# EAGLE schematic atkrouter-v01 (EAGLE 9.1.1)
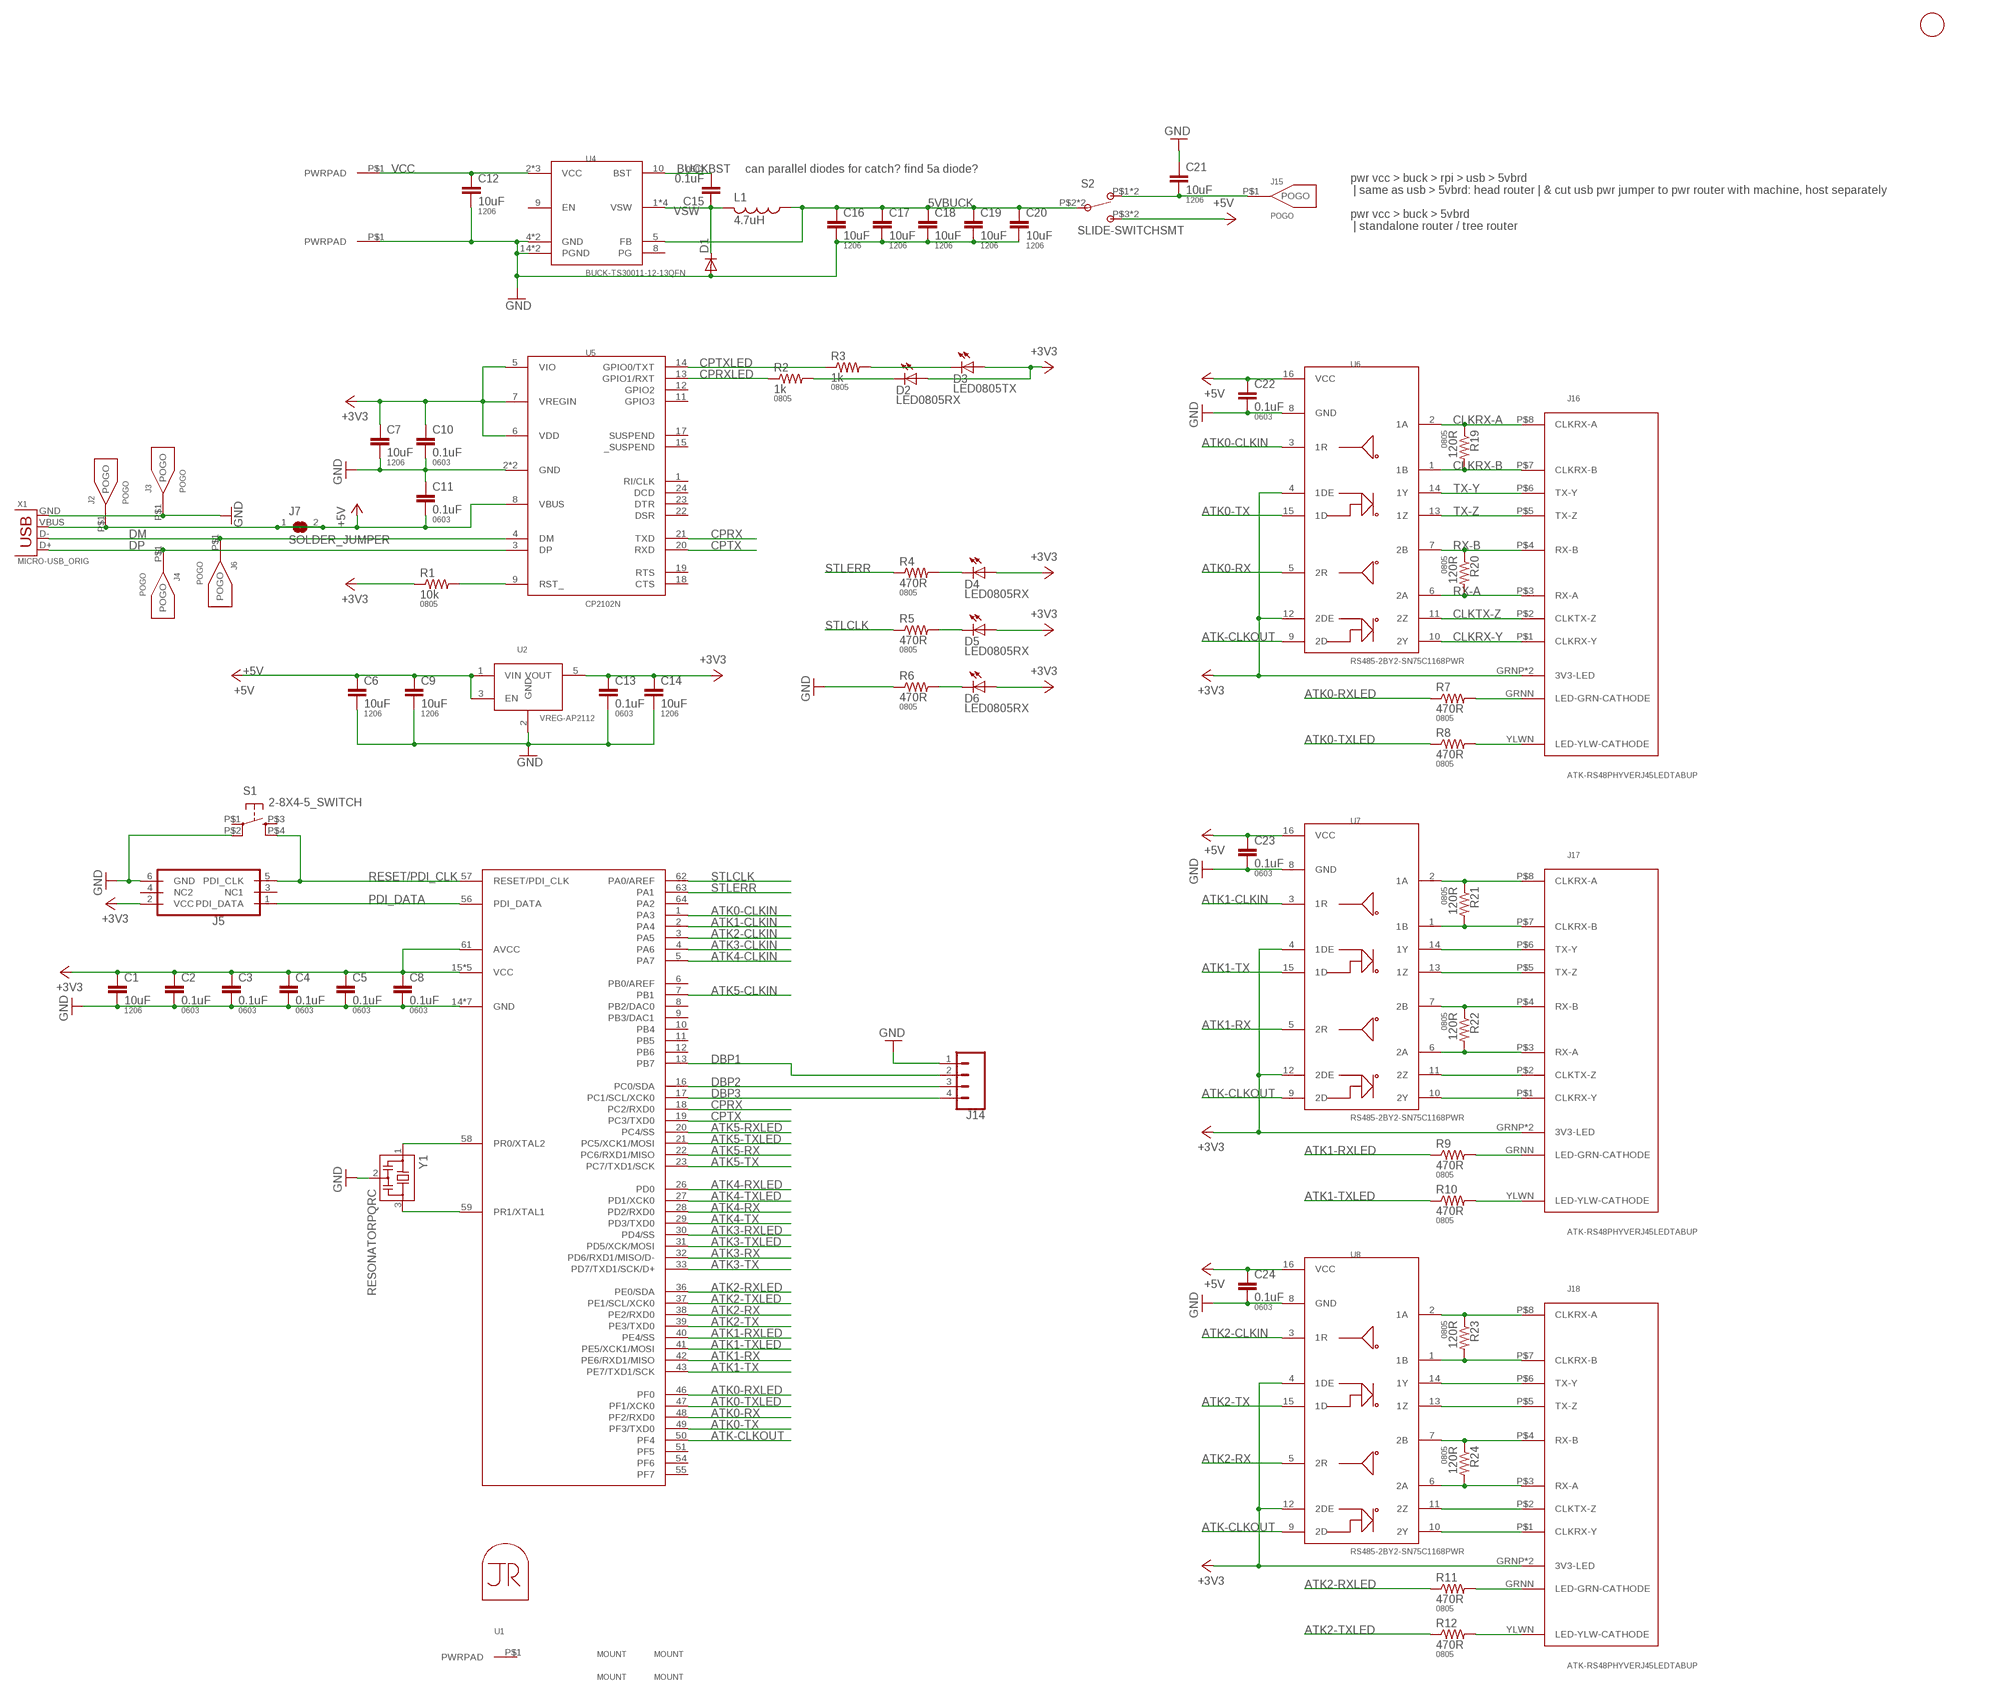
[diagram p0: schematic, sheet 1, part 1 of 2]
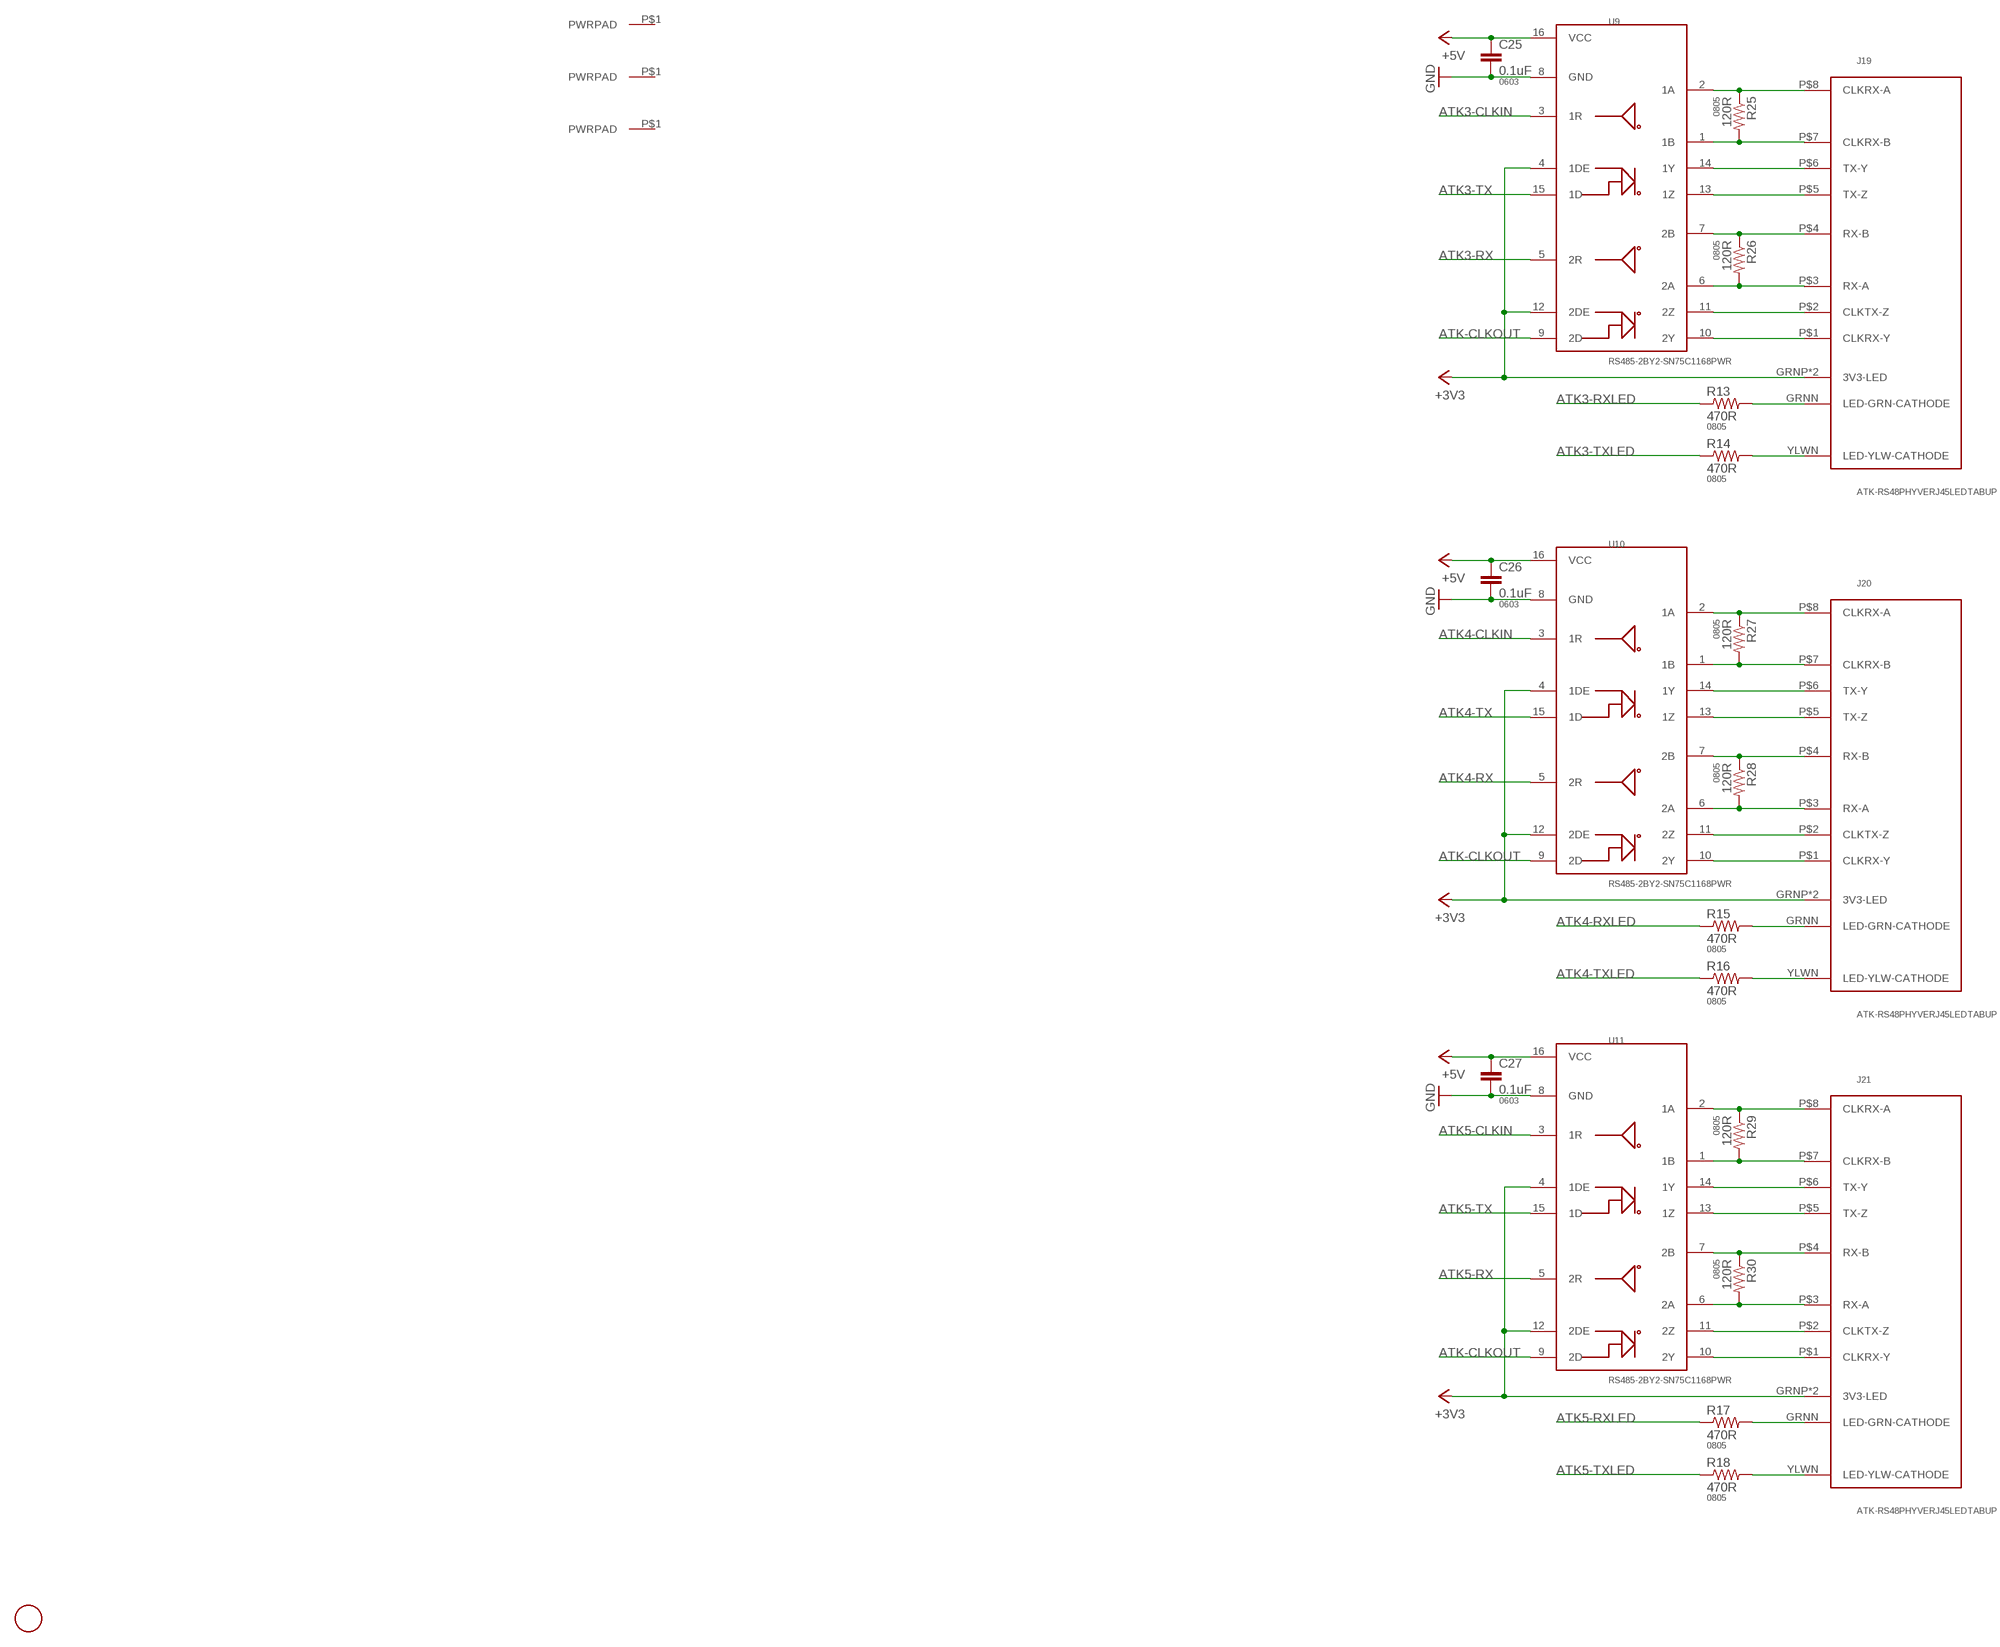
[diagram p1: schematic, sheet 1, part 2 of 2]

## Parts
C1  10uF  CAP1206  [1206]
C2  0.1uF  CAP0603-CAP  [0603-CAP]
C3  0.1uF  CAP0603-CAP  [0603-CAP]
C4  0.1uF  CAP0603-CAP  [0603-CAP]
C5  0.1uF  CAP0603-CAP  [0603-CAP]
C6  10uF  CAP1206  [1206]
C7  10uF  CAP1206  [1206]
C8  0.1uF  CAP0603-CAP  [0603-CAP]
C9  10uF  CAP1206  [1206]
C10  0.1uF  CAP0603-CAP  [0603-CAP]
C11  0.1uF  CAP0603-CAP  [0603-CAP]
C12  10uF  CAP1206  [1206]
C13  0.1uF  CAP0603-CAP  [0603-CAP]
C14  10uF  CAP1206  [1206]
C15  0.1uF  CAP0603-CAP  [0603-CAP]
C16  10uF  CAP1206  [1206]
C17  10uF  CAP1206  [1206]
C18  10uF  CAP1206  [1206]
C19  10uF  CAP1206  [1206]
C20  10uF  CAP1206  [1206]
C21  10uF  CAP1206  [1206]
C22  0.1uF  CAP0603-CAP  [0603-CAP]
C23  0.1uF  CAP0603-CAP  [0603-CAP]
C24  0.1uF  CAP0603-CAP  [0603-CAP]
C25  0.1uF  CAP0603-CAP  [0603-CAP]
C26  0.1uF  CAP0603-CAP  [0603-CAP]
C27  0.1uF  CAP0603-CAP  [0603-CAP]
D1  DIODESOD123HE  [SOD-123HE]
D2  LED0805RX  LED0805  [LED0805]
D3  LED0805TX  LED0805  [LED0805]
D4  LED0805RX  LED0805  [LED0805]
D5  LED0805RX  LED0805  [LED0805]
D6  LED0805RX  LED0805  [LED0805]
J1  FIDUCIAL  [FIDUCIAL_1MM]
J2  POGO  [POGO]
J3  POGO  [POGO]
J4  POGO  [POGO]
J5  PDIFEMALE_SMD  [PDI_2X3_SMD]
J6  POGO  [POGO]
J7  SOLDER_JUMPER  [SJFAB]
J8  PWRPADM3-STANDOFF  [PWRPAD_M3_STANDOFF]
J9  PWRPADM3-STANDOFF  [PWRPAD_M3_STANDOFF]
J10  PWRPADM2.5_STANDOFF  [PWRPAD_M25_STANDOFF]
J11  PWRPADM2.5_STANDOFF  [PWRPAD_M25_STANDOFF]
J12  PWRPADM2.5_STANDOFF  [PWRPAD_M25_STANDOFF]
J13  PWRPADM2.5_STANDOFF  [PWRPAD_M25_STANDOFF]
J14  CONN_041X04_NO_SILK  [1X04_NO_SILK]
J15  POGO  [POGO]
J16  ATK-RS48PHYVERJ45LEDTABUP  [RJ45-LED-RJHSE-5381-UPTAB]
J17  ATK-RS48PHYVERJ45LEDTABUP  [RJ45-LED-RJHSE-5381-UPTAB]
J18  ATK-RS48PHYVERJ45LEDTABUP  [RJ45-LED-RJHSE-5381-UPTAB]
J19  ATK-RS48PHYVERJ45LEDTABUP  [RJ45-LED-RJHSE-5381-UPTAB]
J20  ATK-RS48PHYVERJ45LEDTABUP  [RJ45-LED-RJHSE-5381-UPTAB]
J21  ATK-RS48PHYVERJ45LEDTABUP  [RJ45-LED-RJHSE-5381-UPTAB]
J22  FIDUCIAL  [FIDUCIAL_1MM]
L1  4.7uH  INDUCTOR  [NRS5020T4R7MMGJ]
M1  M3-NPTH  [NPTH-3-25MM]
M2  M3-NPTH  [NPTH-3-25MM]
M3  M3-NPTH  [NPTH-3-25MM]
M4  M3-NPTH  [NPTH-3-25MM]
MP1  JRTOMBSTONE  [JRTOMBSTONE]
R1  10k  RESISTOR0805-RES  [0805]
R2  1k  RESISTOR0805-RES  [0805]
R3  1k  RESISTOR0805-RES  [0805]
R4  470R  RESISTOR0805-RES  [0805]
R5  470R  RESISTOR0805-RES  [0805]
R6  470R  RESISTOR0805-RES  [0805]
R7  470R  RESISTOR0805-RES  [0805]
R8  470R  RESISTOR0805-RES  [0805]
R9  470R  RESISTOR0805-RES  [0805]
R10  470R  RESISTOR0805-RES  [0805]
R11  470R  RESISTOR0805-RES  [0805]
R12  470R  RESISTOR0805-RES  [0805]
R13  470R  RESISTOR0805-RES  [0805]
R14  470R  RESISTOR0805-RES  [0805]
R15  470R  RESISTOR0805-RES  [0805]
R16  470R  RESISTOR0805-RES  [0805]
R17  470R  RESISTOR0805-RES  [0805]
R18  470R  RESISTOR0805-RES  [0805]
R19  120R  RESISTOR0805-RES  [0805]
R20  120R  RESISTOR0805-RES  [0805]
R21  120R  RESISTOR0805-RES  [0805]
R22  120R  RESISTOR0805-RES  [0805]
R23  120R  RESISTOR0805-RES  [0805]
R24  120R  RESISTOR0805-RES  [0805]
R25  120R  RESISTOR0805-RES  [0805]
R26  120R  RESISTOR0805-RES  [0805]
R27  120R  RESISTOR0805-RES  [0805]
R28  120R  RESISTOR0805-RES  [0805]
R29  120R  RESISTOR0805-RES  [0805]
R30  120R  RESISTOR0805-RES  [0805]
S1  2-8X4-5_SWITCH  [TACT-SWITCH-KMR6]
S2  SLIDE-SWITCHSMT  [SLIDESWITCH-CL-SB-22A]
U1  RASPBERRYPI-3BPLUS  [RASPBERRYPI-3BPLUS]
U2  VREG-AP2112  [SOT23-5]
U3  ATXMEGA_A3UQFN  [QFN-64-9X9MM]
U4  BUCK-TS30011-12-13QFN  [QFN16-3X3-TI-RTE]
U5  CP2102N  [QFN-24_ALT2]
U6  RS485-2BY2-SN75C1168PWR  [TSSOP16]
U7  RS485-2BY2-SN75C1168PWR  [TSSOP16]
U8  RS485-2BY2-SN75C1168PWR  [TSSOP16]
U9  RS485-2BY2-SN75C1168PWR  [TSSOP16]
U10  RS485-2BY2-SN75C1168PWR  [TSSOP16]
U11  RS485-2BY2-SN75C1168PWR  [TSSOP16]
X1  MICRO-USB_ORIG  [DX4R005HJ5]
Y1  RESONATORPQRC  [RES_PRQC]

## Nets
5VBUCK: C16.1 C17.1 C18.1 C19.1 C20.1 L1.1 S2.P$2 S2.P$5 U4.5(FB)
+3V3: C1.1 C2.1 C3.1 C4.1 C5.1 C7.1 C8.1 C10.1 C13.1 C14.1 D2.1(A) D3.1(A) D4.1(A) D5.1(A) D6.1(A) J5.2(VCC) J16.GRNP(3V3-LED) J16.YLWP(3V3-LED) J17.GRNP(3V3-LED) J17.YLWP(3V3-LED) J18.GRNP(3V3-LED) J18.YLWP(3V3-LED) J19.GRNP(3V3-LED) J19.YLWP(3V3-LED) J20.GRNP(3V3-LED) J20.YLWP(3V3-LED) J21.GRNP(3V3-LED) J21.YLWP(3V3-LED) R1.1 U2.5(VOUT) U3.15(VCC) U3.25(VCC) U3.35(VCC) U3.45(VCC) U3.53(VCC) U3.61(AVCC) U5.5(VIO) U5.6(VDD) U5.7(VREGIN) U6.4(1DE) U6.12(2DE) U7.4(1DE) U7.12(2DE) U8.4(1DE) U8.12(2DE) U9.4(1DE) U9.12(2DE) U10.4(1DE) U10.12(2DE) U11.4(1DE) U11.12(2DE)
+5V: C6.1 C9.1 C11.2 C22.1 C23.1 C24.1 C25.1 C26.1 C27.1 J2.P$1(POGO) J7.1 J7.2 S2.P$3 S2.P$6 U2.1(VIN) U2.3(EN) U5.8(VBUS) U6.16(VCC) U7.16(VCC) U8.16(VCC) U9.16(VCC) U10.16(VCC) U11.16(VCC) X1.VBUS
ATK0-CLKIN: U3.1(PA3) U6.3(1R)
ATK0-RX: U3.48(PF2/RXD0) U6.5(2R)
ATK0-RXLED: R7.1 U3.46(PF0)
ATK0-TX: U3.49(PF3/TXD0) U6.15(1D)
ATK0-TXLED: R8.1 U3.47(PF1/XCK0)
ATK1-CLKIN: U3.2(PA4) U7.3(1R)
ATK1-RX: U3.42(PE6/RXD1/MISO) U7.5(2R)
ATK1-RXLED: R9.1 U3.40(PE4/SS)
ATK1-TX: U3.43(PE7/TXD1/SCK) U7.15(1D)
ATK1-TXLED: R10.1 U3.41(PE5/XCK1/MOSI)
ATK2-CLKIN: U3.3(PA5) U8.3(1R)
ATK2-RX: U3.38(PE2/RXD0) U8.5(2R)
ATK2-RXLED: R11.1 U3.36(PE0/SDA)
ATK2-TX: U3.39(PE3/TXD0) U8.15(1D)
ATK2-TXLED: R12.1 U3.37(PE1/SCL/XCK0)
ATK3-CLKIN: U3.4(PA6) U9.3(1R)
ATK3-RX: U3.32(PD6/RXD1/MISO/D-) U9.5(2R)
ATK3-RXLED: R13.1 U3.30(PD4/SS)
ATK3-TX: U3.33(PD7/TXD1/SCK/D+) U9.15(1D)
ATK3-TXLED: R14.1 U3.31(PD5/XCK/MOSI)
ATK4-CLKIN: U3.5(PA7) U10.3(1R)
ATK4-RX: U3.28(PD2/RXD0) U10.5(2R)
ATK4-RXLED: R15.1 U3.26(PD0)
ATK4-TX: U3.29(PD3/TXD0) U10.15(1D)
ATK4-TXLED: R16.1 U3.27(PD1/XCK0)
ATK5-CLKIN: U3.7(PB1) U11.3(1R)
ATK5-RX: U3.22(PC6/RXD1/MISO) U11.5(2R)
ATK5-RXLED: R17.1 U3.20(PC4/SS)
ATK5-TX: U3.23(PC7/TXD1/SCK) U11.15(1D)
ATK5-TXLED: R18.1 U3.21(PC5/XCK1/MOSI)
ATK-CLKOUT: U3.50(PF4) U6.9(2D) U7.9(2D) U8.9(2D) U9.9(2D) U10.9(2D) U11.9(2D)
BUCKBST: C15.2 U4.10(BST)
CLKRX-A: J16.P$8(CLKRX-A) R19.1 U6.2(1A)
CLKRX-B: J16.P$7(CLKRX-B) R19.2 U6.1(1B)
CLKRX-Y: J16.P$1(CLKRX-Y) U6.10(2Y)
CLKTX-Z: J16.P$2(CLKTX-Z) U6.11(2Z)
CPRX: U3.18(PC2/RXD0) U5.21(TXD)
CPRXLED: R2.1 U5.13(GPIO1/RXT)
CPTX: U3.19(PC3/TXD0) U5.20(RXD)
CPTXLED: R3.1 U5.14(GPIO0/TXT)
DBP1: J14.2 U3.13(PB7)
DBP2: J14.3 U3.16(PC0/SDA)
DBP3: J14.4 U3.17(PC1/SCL/XCK0)
DM: J6.P$1(POGO) U5.4(DM) X1.D-
DP: J4.P$1(POGO) U5.3(DP) X1.D+
GND: C1.2 C2.2 C3.2 C4.2 C5.2 C6.2 C7.2 C8.2 C9.2 C10.2 C11.1 C12.2 C13.2 C14.2 C16.2 C17.2 C18.2 C19.2 C20.2 C21.1 C22.2 C23.2 C24.2 C25.2 C26.2 C27.2 D1.P$2(A) J3.P$1(POGO) J5.6(GND) J9.P$1(PWRPAD) J14.1 R6.1 S1.P$2(P1) U2.2(GND) U3.14(GND) U3.24(GND) U3.34(GND) U3.44(GND) U3.52(GND) U3.60(GND) U3.P$1(GND) U4.4(GND) U4.14(PGND) U4.15(PGND) U4.TH(GND) U5.2(GND) U5.EP(GND) U6.8(GND) U7.8(GND) U8.8(GND) U9.8(GND) U10.8(GND) U11.8(GND) X1.GND Y1.2
N$1: J16.GRNN(LED-GRN-CATHODE) R7.2
N$2: J16.YLWN(LED-YLW-CATHODE) R8.2
N$3: J18.P$6(TX-Y) U8.14(1Y)
N$4: J18.P$5(TX-Z) U8.13(1Z)
N$5: J18.P$4(RX-B) R24.1 U8.7(2B)
N$6: J18.P$3(RX-A) R24.2 U8.6(2A)
N$7: J18.P$8(CLKRX-A) R23.1 U8.2(1A)
N$8: J18.P$7(CLKRX-B) R23.2 U8.1(1B)
N$9: J18.P$2(CLKTX-Z) U8.11(2Z)
N$10: J18.P$1(CLKRX-Y) U8.10(2Y)
N$13: U3.58(PR0/XTAL2) Y1.1
N$14: U3.59(PR1/XTAL1) Y1.3
N$15: D6.2(C) R6.2
N$17: D5.2(C) R5.2
N$19: R1.2 U5.9(RST_)
N$21: D4.2(C) R4.2
N$25: J17.P$6(TX-Y) U7.14(1Y)
N$26: J17.P$5(TX-Z) U7.13(1Z)
N$27: J17.P$4(RX-B) R22.1 U7.7(2B)
N$28: J17.P$3(RX-A) R22.2 U7.6(2A)
N$29: J17.P$8(CLKRX-A) R21.1 U7.2(1A)
N$30: J17.P$7(CLKRX-B) R21.2 U7.1(1B)
N$31: J17.P$2(CLKTX-Z) U7.11(2Z)
N$32: J17.P$1(CLKRX-Y) U7.10(2Y)
N$33: J17.GRNN(LED-GRN-CATHODE) R9.2
N$34: J17.YLWN(LED-YLW-CATHODE) R10.2
N$35: J18.GRNN(LED-GRN-CATHODE) R11.2
N$36: J18.YLWN(LED-YLW-CATHODE) R12.2
N$37: D2.2(C) R2.2
N$38: D3.2(C) R3.2
N$39: J19.P$6(TX-Y) U9.14(1Y)
N$40: J19.P$5(TX-Z) U9.13(1Z)
N$41: J19.P$4(RX-B) R26.1 U9.7(2B)
N$42: J19.P$3(RX-A) R26.2 U9.6(2A)
N$43: J19.P$8(CLKRX-A) R25.1 U9.2(1A)
N$44: J19.P$7(CLKRX-B) R25.2 U9.1(1B)
N$45: J19.P$2(CLKTX-Z) U9.11(2Z)
N$46: J19.P$1(CLKRX-Y) U9.10(2Y)
N$47: J19.GRNN(LED-GRN-CATHODE) R13.2
N$48: J19.YLWN(LED-YLW-CATHODE) R14.2
N$49: J20.P$6(TX-Y) U10.14(1Y)
N$50: J20.P$5(TX-Z) U10.13(1Z)
N$51: J20.P$4(RX-B) R28.1 U10.7(2B)
N$52: J20.P$3(RX-A) R28.2 U10.6(2A)
N$53: J20.P$8(CLKRX-A) R27.1 U10.2(1A)
N$54: J20.P$7(CLKRX-B) R27.2 U10.1(1B)
N$55: J20.P$2(CLKTX-Z) U10.11(2Z)
N$56: J20.P$1(CLKRX-Y) U10.10(2Y)
N$57: J20.GRNN(LED-GRN-CATHODE) R15.2
N$58: J20.YLWN(LED-YLW-CATHODE) R16.2
N$59: J21.P$6(TX-Y) U11.14(1Y)
N$60: J21.P$5(TX-Z) U11.13(1Z)
N$61: J21.P$4(RX-B) R30.1 U11.7(2B)
N$62: J21.P$3(RX-A) R30.2 U11.6(2A)
N$63: J21.P$8(CLKRX-A) R29.1 U11.2(1A)
N$64: J21.P$7(CLKRX-B) R29.2 U11.1(1B)
N$65: J21.P$2(CLKTX-Z) U11.11(2Z)
N$66: J21.P$1(CLKRX-Y) U11.10(2Y)
N$67: J21.GRNN(LED-GRN-CATHODE) R17.2
N$68: J21.YLWN(LED-YLW-CATHODE) R18.2
N$69: C21.2 J15.P$1(POGO) S2.P$1 S2.P$4
PDI_DATA: J5.1(PDI_DATA) U3.56(PDI_DATA)
RESET/PDI_CLK: J5.5(PDI_CLK) S1.P$4(S1) U3.57(RESET/PDI_CLK)
RX-A: J16.P$3(RX-A) R20.2 U6.6(2A)
RX-B: J16.P$4(RX-B) R20.1 U6.7(2B)
STLCLK: R5.1 U3.62(PA0/AREF)
STLERR: R4.1 U3.63(PA1)
TX-Y: J16.P$6(TX-Y) U6.14(1Y)
TX-Z: J16.P$5(TX-Z) U6.13(1Z)
VCC: C12.1 J8.P$1(PWRPAD) U4.2(VCC) U4.3(VCC) U4.11(VCC)
VSW: C15.1 D1.P$1(C) L1.2 U4.1(VSW) U4.12(VSW) U4.13(VSW) U4.16(VSW)
Unconnected: J5.3(NC1) J5.4(NC2) J10.P$1(PWRPAD) J11.P$1(PWRPAD) J12.P$1(PWRPAD) J13.P$1(PWRPAD) S1.P$1(P) S1.P$3(S) U3.6(PB0/AREF) U3.8(PB2/DAC0) U3.9(PB3/DAC1) U3.10(PB4) U3.11(PB5) U3.12(PB6) U3.51(PF5) U3.54(PF6) U3.55(PF7) U3.64(PA2) U4.8(PG) U4.9(EN) U5.1(RI/CLK) U5.11(GPIO3) U5.12(GPIO2) U5.15(_SUSPEND) U5.17(SUSPEND) U5.18(CTS) U5.19(RTS) U5.22(DSR) U5.23(DTR) U5.24(DCD)

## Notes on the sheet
- can parallel diodes for catch? find 5a diode?
- pwr vcc > buck > rpi > usb > 5vbrd
   | same as usb > 5vbrd: head router | & cut usb pwr jumper to pwr router with machine, host separately
  
  pwr vcc > buck > 5vbrd
   | standalone router / tree router

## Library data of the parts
C1 C6 C7 C9 C12 C14 C16-C21 = passives:CAP: Capacitor; PACKAGE: 1206
C2-C5 C8 C10 C11 C13 C15 C22-C27 = passives:CAP: Capacitor; PACKAGE: 0603
D1 = passives:DIODE: DIODE
D2-D6 = lights:LED: LED
J1 J22 = connector:FIDUCIAL: For use by pick and place machines to calibrate the vision/machine, 1mm
J2-J4 J6 J15 = connector:POGO
J5 = microcontrollers:PDI: Multi connection point. Often used as Generic Header-pin footprint for 0.1 inch spaced/style header connections You can populate with any combo of single row headers, but if you'd like an exact match, check these: Header - 2x3 (Male, 0.1") (PRT-12807) Header - 2x3 (Female, 0.1") (PRT-13010) 2x3 Pin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; PROD_ID: CONN-11290
J7 = connector:SOLDER_JUMPER
J8-J13 = power:PWRPAD
J14 = SparkFun-Connectors:CONN_04: Multi connection point. Often used as Generic Header-pin footprint for 0.1 inch spaced/style header connections On any of the 0.1 inch spaced packages, you can populate with these: Break Away Headers - Straight (PRT-00116) Break Away Male Headers - Right Angle (PRT-00553) Female Headers (PRT-00115)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; PROD_ID: CONN-09696
J16-J21 = connector:ATK-RS48PHYVE
L1 = power:INDUCTOR
M1-M4 = power:M3-NPTH
MP1 = connector:JRTOMBSTONE
R1-R30 = passives:RESISTOR: Resistor; PACKAGE: 0805
S1 = passives:2-8X4-5_SWITCH
S2 = fab:SLIDE-SWITCH: SMD slide-switch AYZ0102AGRLC as found in the fablab inventory. Includes the mounting holes. Made by Zaerc.
U1 = connector:RASPBERRYPI-3BPLUS
U2 = power:VREG-AP2112
U3 = microcontrollers:ATXMEGA_A3U
U4 = power:BUCK-TS30011-12-13
U5 = microcontrollers:CP2102N
U6-U11 = comm:RS485-2BY2-SN75C1168PWR
X1 = connector:MICRO-USB: SMD micro USB connector as found in the fablab inventory. Three footprint variants included: original, as described by manufacturer's datasheet for milling with the 1/100" bit for milling with the 1/64" bit Made by Zaerc.
Y1 = passives:RESONATOR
